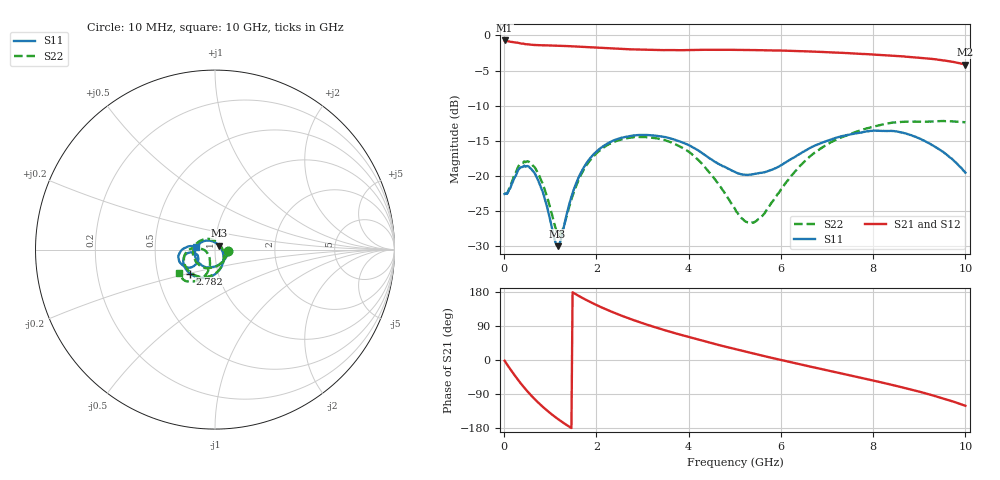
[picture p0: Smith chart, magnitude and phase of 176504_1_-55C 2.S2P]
!  2-Port S-parameters saved by WinCal
! VAR MeasName=S-Parameters (CALIBRATED_DATA) read from VNA (N5242A)
! VAR MeasDate=2017-11-2 17:07:14
! VAR NAME=176504_1_-55C 2
! VAR FILENAME=176504_1_-55C 2.S2P
! VAR DATE=2017-11-2 17:07:14
! VAR PHYS_PORTS=2,3
# Hz S DB R 50
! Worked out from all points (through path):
!   401 points, 10 MHz to 10 GHz, reference 50 ohm
!   highest |S21| = -0.71 dB at 10 MHz (marker M1); lowest = -4.2 dB at 10 GHz (marker M2)
!   lowest |S11| = -30.0 dB at 1.159 GHz (marker M3), VSWR 1.07, Z = 52.3 + j2.22 ohm
!   |S11| at or under -10 dB: start of sweep to end of sweep
!   |S22| runs from -28.4 to -12.2 dB; largest |S21 - S12| = 0.0082
!   S11 on the Smith chart (normalised r, x): 10 MHz: 1.16, -0.02; 2.782 GHz: 0.73, -0.20; 10 GHz: 0.81, +0.02
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1e7  -22.59 -5.4  -0.71 -2.1  -0.71 -2.1  -22.58 -5.6
1.34875e8  -21.74 -66.1  -0.89 -24.5  -0.89 -24.5  -21.53 -68.5
2.5975e8  -19.88 -104.7  -1.02 -45.6  -1.02 -45.6  -19.44 -107.0
4.84525e8  -18.62 -155.9  -1.25 -79.9  -1.26 -79.9  -17.97 -157.8
6.34375e8  -19.39 177.3  -1.34 -99.8  -1.34 -99.8  -18.61 175.3
8.34175e8  -22.22 142.2  -1.40 -123.2  -1.40 -123.2  -21.08 140.5
1.15885e9  -30.03 42.2  -1.46 -155.1  -1.45 -155.1  -28.18 52.9
1.25875e9  -28.33 -2.7  -1.48 -163.6  -1.48 -163.9  -27.85 10.5
1.45855e9  -22.99 -47.8  -1.54 -179.5  -1.54 -179.5  -23.36 -42.2
1.683325e9  -19.32 -73.4  -1.62 164.6  -1.62 164.7  -19.64 -71.2
2.182825e9  -15.64 -108.1  -1.80 135.0  -1.81 135.0  -15.86 -108.8
2.782225e9  -14.28 -136.3  -1.98 106.3  -1.99 106.4  -14.52 -139.3
3.35665e9  -14.36 -156.3  -2.07 83.2  -2.09 83.3  -14.74 -161.1
4.15585e9  -16.19 -172.5  -2.06 55.6  -2.07 55.7  -17.40 178.1
5.005e9  -19.46 -166.1  -2.05 28.8  -2.04 28.8  -24.72 -176.6
5.279725e9  -19.88 -159.0  -2.07 20.6  -2.07 20.7  -26.63 -154.7
5.5045e9  -19.66 -153.7  -2.09 14.0  -2.09 14.2  -26.20 -133.9
6.678325e9  -15.86 -142.8  -2.29 -18.5  -2.31 -18.4  -16.97 -109.0
7.577425e9  -14.02 -153.7  -2.57 -42.7  -2.59 -42.6  -13.86 -121.1
8.35165e9  -13.62 -167.2  -2.85 -64.0  -2.90 -64.0  -12.49 -131.8
9.25075e9  -15.50 176.8  -3.32 -91.9  -3.34 -91.5  -12.28 -140.7
1e10  -19.56 172.3  -4.15 -120.8  -4.16 -120.4  -12.37 -147.5
